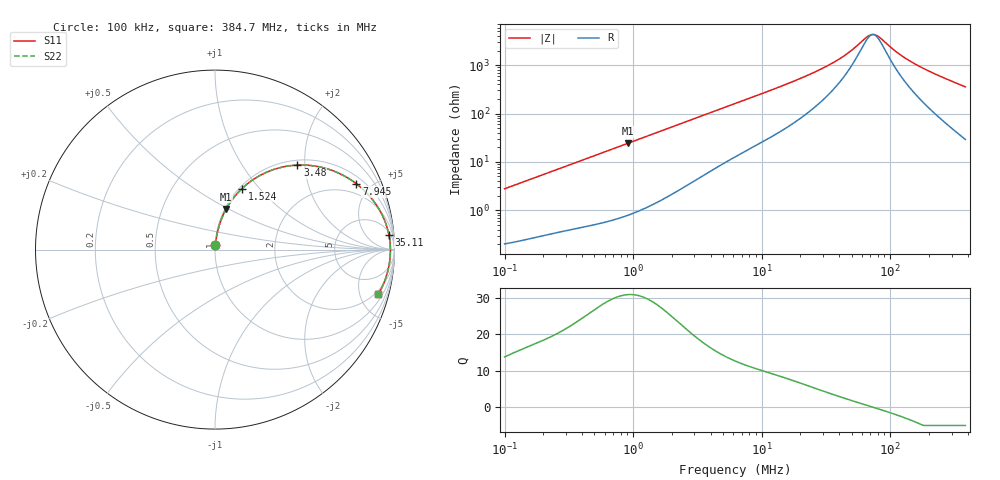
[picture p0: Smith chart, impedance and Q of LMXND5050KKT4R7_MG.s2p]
! LMXND5050KKT4R7_MG  S-PARAMETER MODEL  ( General Type )
! Model Generated by TAIYO YUDEN Corporation (http://www.ty-top.com)
! Version 1.0
! TAIYO YUDEN Control No. 191023NI43SB-FBB
! Copyright(c) 2019 TAIYO YUDEN CO.,LTD. All Rights Reserved.
! Product Description (link to TY-COMPAS)
! https://ds.yuden.co.jp/TYCOMPAS/or/detail?pn=LMXND5050KKT4R7MMG&u=M
! Products Name : Inductors
! Characteristics :
!  Inductance : 4.7 uH , SRF(min) : 37 MHz , DC Resistance(max) : 0.174 Ohm
!  Rated Current : Saturation :1200 mA , Temp Rise : 1150 mA
!  Case Size : 4.9 x 4.9 / 0.193 x 0.193 [mm/inch] , Thickness : 1 / 0.039 [mm/inch]
!  (Conditions: Temperature = 25 degC , DC Bias Current/Voltage = 0A / 0V)
! External Node Assignments :
!  1  o---GGG---o  2
! GND o---------o GND
! Frequency Range : 0.1MHz  -  384.651195MHz  [ 402 STEP ]
# MHz S RI R 50
! Freq[MHz].  S11 Real  S11 Imag  S21 Real  S21 Imag  S12 Real  S12 Imag  S22 Real  S22 Imag
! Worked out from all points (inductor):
!   401 points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, 100 kHz to 384.7 MHz, reference 50 ohm
!   read as one part in series: L = 4.4 uH near 104.2 kHz
!   highest Q = 30.8 at 909.9 kHz (marker M1), where L = 4.25 uH
!   self-resonance near 73.36 MHz
!   S11 on the Smith chart (normalised r, x): 100 kHz: 1.00, +0.06; 1.524 MHz: 1.03, +0.81; 3.48 MHz: 1.10, +1.83; 7.945 MHz: 1.36, +4.08; 35.11 MHz: 7, +21; 384.7 MHz: 1.58, -7.11
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0.1  0.00278 0.0276  0.9972 -0.0276  0.9972 -0.0276  0.00278 0.0276
0.398565  0.0157 0.1053  0.9843 -0.1053  0.9843 -0.1053  0.0157 0.1053
0.909925  0.0623 0.2261  0.9377 -0.2261  0.9377 -0.2261  0.0623 0.2261
1.524306  0.15 0.3398  0.85 -0.3398  0.85 -0.3398  0.15 0.3398
1.588538  0.1604 0.3494  0.8396 -0.3494  0.8396 -0.3494  0.1604 0.3494
2.256123  0.2723 0.4241  0.7277 -0.4241  0.7277 -0.4241  0.2723 0.4241
3.479997  0.4588 0.4709  0.5412 -0.4709  0.5412 -0.4709  0.4588 0.4709
6.331348  0.7143 0.4136  0.2857 -0.4136  0.2857 -0.4136  0.7143 0.4136
7.944847  0.7876 0.3669  0.2124 -0.3669  0.2124 -0.3669  0.7876 0.3669
13.30921  0.8975 0.2512  0.1025 -0.2512  0.1025 -0.2512  0.8975 0.2512
24.71908  0.9553 0.1345  0.0447 -0.1345  0.0447 -0.1345  0.9553 0.1345
35.10732  0.9687 0.0839  0.0313 -0.0839  0.0313 -0.0839  0.9687 0.0839
45.91053  0.974 0.051  0.026 -0.051  0.026 -0.051  0.974 0.051
65.20451  0.9771 0.0125  0.0229 -0.0125  0.0229 -0.0125  0.9771 0.0125
70.8155  0.9773 0.00373  0.0227 -0.00373  0.0227 -0.00373  0.9773 0.00373
75.33839  0.9774 -0.00281  0.0226 0.00281  0.0226 0.00281  0.9774 -0.00281
80.15015  0.9773 -0.00936  0.0227 0.00936  0.0227 0.00936  0.9773 -0.00936
98.5215  0.9765 -0.0316  0.0235 0.0316  0.0235 0.0316  0.9765 -0.0316
126.2069  0.9739 -0.06  0.0261 0.06  0.0261 0.06  0.9739 -0.06
168.4847  0.9679 -0.0974  0.0321 0.0974  0.0321 0.0974  0.9679 -0.0974
249.3739  0.9509 -0.1597  0.0491 0.1597  0.0491 0.1597  0.9509 -0.1597
384.6512  0.9098 -0.2485  0.0902 0.2485  0.0902 0.2485  0.9098 -0.2485
